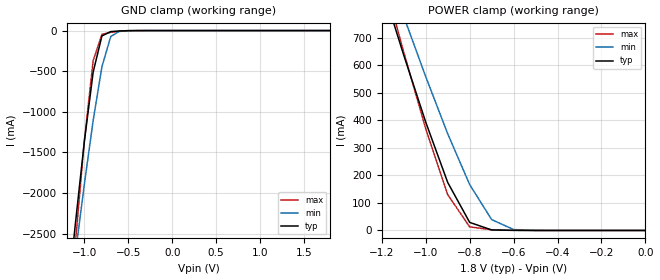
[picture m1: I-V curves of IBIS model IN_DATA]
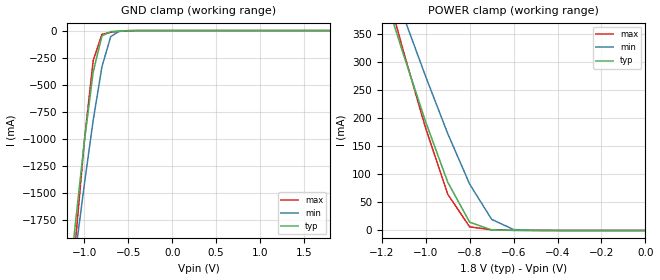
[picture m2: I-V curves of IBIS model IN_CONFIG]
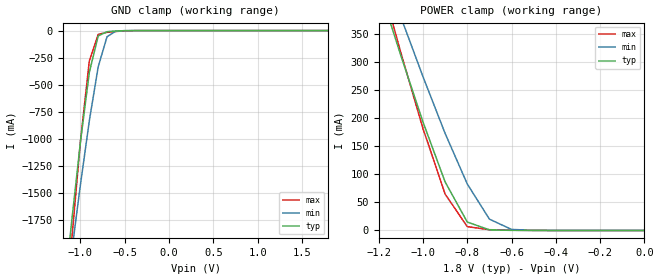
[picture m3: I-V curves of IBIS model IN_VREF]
| IBIS file 4pw864dy_ab_t.ibs created by s2ibis2 version 1.2
| North Carolina State University Electronics Research Laboratory  1995
[IBIS ver]   2.1
[File name]   4pw864dy_ab_t.ibs
[File Rev]   1.0
[Date]   Friday, March 12, 2004
[Source]   IDT
[Notes]   1. Temp typ=25C, min=0C, max=110C
   2. IDT C11.5 1.8V 1P 2-6M process
   3. Ramp rates based on 10Gig ohm load
   *** Important Notes ***
This IBIS file is for the 1:2 Registered Buffer with configuration settings
c0=0, c1=1 (Type A) and c0=1, c1=1 (Type B)
[Disclaimer]
READ THESE TERMS AND CONDITIONS CAREFULLY BEFORE USING THIS IBIS MODEL.  BY
USING THIS IBIS MODEL, YOU ARE ACCEPTING AND AGREEING TO THESE TERMS AND
CONDITIONS OF USE.
Integrated Device Technology, Inc. ("IDT") hereby grants the user of this
IBIS model ("User") a non-exclusive, nontransferable license to use this
IBIS model under the following terms: The User is granted this license only
to use the IBIS model for demonstration purposes only and is not granted
rights to sell, copy (except as needed to run the IBIS model), rent, lease
or sub-license (except for demonstration) the IBIS model in whole or in
part, or in modified form to anyone. The User may modify the IBIS model to
suit its specific applications, but  rights to derivative works and such
modifications shall belong to IDT.
THIS IBIS MODEL IS PROVIDED ON AN AS IS" BASIS AND IDT  MAKES ABSOLUTELY NO
WARRANTY WITH RESPECT TO THE INFORMATION CONTAINED HEREIN.  IDT DISCLAIMS
AND USER WAIVES ALL WARRANTIES, EXPRESS AND IMPLIED, INCLUDING WARRANTIES OF
MERCHANTABILITY AND FITNESS FOR A PARTICULAR PURPOSE.  THE ENTIRE RISK AS TO
QUALITY AND PERFORMANCE IS WITH THE USER  ACCORDINGLY, IN NO EVENT SHALL IDT
BE LIABLE FOR ANY DIRECT OR INDIRECT DAMAGES, WHETHER IN CONTRACT OR TORT,
INCLUDING ANY LOST PROFITS OR OTHER INCIDENTAL, CONSEQUENTIAL, EXEMPLARY, OR
PUNITIVE DAMAGES ARISING OUT OF THE USE OR APPLICATION OF THE  IBIS MODEL,
WHETHER OR NOT IDT HAD NOTICE OF SUCH DAMAGES.
IDT reserves the right to make changes without notice to any product herein
to improve reliability, function, or design. IDT does not convey any license
under patent rights or any other intellectual property rights, including
those of third parties. IDT is not obligated to provide  maintenance or
support for the licensed IBIS model.
This model is IDT74SSTU32864C 1:2 Registered Buffer with 1.8 SSTL I/O
[Copyright]
Copyright 2002, Integrated Device Technology, Inc. All rights
reserved.
|   Component IDT4PW864DY
[Component]   IDT4PW864DY
[Manufacturer]   Integrated Device Technology, Inc.
[Package]
| variable   typ   min   max
R_pkg   0.01480   0.01480   0.01480
L_pkg   1.05000nH   1.05000nH   1.05000nH
C_pkg   0.29100pF   0.29100pF   0.29100pF
[Pin]  signal_name   model_name   R_pin   L_pin   C_pin
A1   DCKE/D1   IN_DATA
A2   NC   NC
A3   VREF   IN_VREF
A4   VDD   POWER
A5   QCKEA/Q1A   OUTBUF
A6   QCKEB/Q1B   OUTBUF
B1   D2   IN_DATA
B2   NC   NC
B3   GND   GND
B4   GND   GND
B5   Q2A   OUTBUF
B6   Q2B   OUTBUF
C1   D3   IN_DATA
C2   NC   NC
C3   VDD   POWER
C4   VDD   POWER
C5   Q3A   OUTBUF
C6   Q3B   OUTBUF
D1   DODT/D4   IN_DATA
D2   NC   NC
D3   GND   GND
D4   GND   GND
D5   QODTA/Q4A   OUTBUF
D6   QODTB/Q4B   OUTBUF
E1   D5   IN_DATA
E2   NC   NC
E3   VDD   POWER
E4   VDD   POWER
E5   Q5A   OUTBUF
E6   Q5B   OUTBUF
F1   D6   IN_DATA
F2   NC   NC
F3   GND   GND
F4   GND   GND
F5   Q6A   OUTBUF
F6   Q6B   OUTBUF
G1   NC   NC
G2   _RESET_   IN_RESET
G3   VDD   POWER
G4   VDD   POWER
G5   C1   IN_CONFIG
G6   C0   IN_CONFIG
H1   CLK   IN_CLK
H2   _DCS_   IN_CSGATEN
H3   GND   GND
H4   GND   GND
H5   _QCSA_   OUTBUF
H6   _QCSB_   OUTBUF
J1   _CLK_   IN_CLK
J2   _CSR_   IN_CSGATEN
J3   VDD   POWER
J4   VDD   POWER
J5   NC   NC
J6   NC   NC
K1   D8   IN_DATA
K2   NC   NC
K3   GND   GND
K4   GND   GND
K5   Q8A   OUTBUF
K6   Q8B   OUTBUF
L1   D9   IN_DATA
L2   NC   NC
L3   VDD   POWER
L4   VDD   POWER
L5   Q9A   OUTBUF
L6   Q9B   OUTBUF
M1   D10   IN_DATA
M2   NC   NC
M3   GND   GND
M4   GND   GND
M5   Q10A   OUTBUF
M6   Q10B   OUTBUF
N1   D11/DODT   IN_DATA
N2   NC   NC
N3   VDD   POWER
N4   VDD   POWER
N5   Q11A/QODTA   OUTBUF
N6   Q11B/QODTB   OUTBUF
P1   D12   IN_DATA
P2   NC   NC
P3   GND   GND
P4   GND   GND
P5   Q12A   OUTBUF
P6   Q12B   OUTBUF
R1   D13   IN_DATA
R2   NC   NC
R3   VDD   POWER
R4   VDD   POWER
R5   Q13A   OUTBUF
R6   Q13B   OUTBUF
T1   D14/DCKE   IN_DATA
T2   NC   NC
T3   VREF   IN_VREF
T4   VDD   POWER
T5   Q14A/QCKEA   OUTBUF
T6   Q14B/QCKEB   OUTBUF
| d   d   dummy_model
| din  din   dummy_model
[Diff Pin]  inv_pin   vdiff   tdelay_typ  tdelay_min  tdelay_max
H1   J1   0.60000V  NA   |CLK<P:N> Input  Pair
| Models and submodels in the file (7): IN_DATA (Input), IN_CONFIG (Input), IN_VREF (Input), IN_CLK (Input), IN_CSGATEN (Input), IN_RESET (Input), OUTBUF (Output)
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|   Model IN_DATA
[Model]   IN_DATA
Model_type   Input
Vinl =  0.65000V
Vinh =  1.15000V
C_comp   2.50000pF   2.50000pF   2.50000pF
[Temperature Range]   25.00000   0.11000k   0.000
[Voltage Range]   1.80000V   1.70000V   1.90000V
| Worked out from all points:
|   GND clamp passes 1 mA (typ) near -0.50 V on its own axis
|   POWER clamp passes 1 mA (typ) near -0.64 V on its own axis
[GND_clamp]
| voltage   I(typ)   I(min)   I(max)
-1.8V     -10.01A    -9.034A    -12.29A
-1.2V     -3.402A    -3.598A    -3.91A
-1.1V     -2.357A    -2.731A    -2.591A
-1V       -1.366A    -1.893A    -1.357A
-900mV    -512.4mA   -1.108A    -371.9mA
-800mV    -65.6mA    -445.2mA   -46.17mA
-700mV    -12.81mA   -74.32mA   -21.4mA
-600mV    -4.632mA   -6.378mA   -10.47mA
-400mV    -151.1uA   -107.5uA   -515.4uA
1.8V      13.82nA    12.76nA    492.7pA
[POWER_clamp]
| voltage   I(typ)   I(min)   I(max)
-1.8V     2.486A     2.403A     2.783A
-1.2V     891mA      1.002A     940.1mA
-1.1V     637mA      777.5mA    647.6mA
-1V       393.6mA    558.9mA    369.7mA
-900mV    174.5mA    351.3mA    130.1mA
-800mV    29.33mA    166.7mA    13.12mA
-700mV    1.951mA    39.57mA    2.484mA
-600mV    305.6uA    3.357mA    798.8uA
-500mV    48.35uA    239.3uA    163.9uA
0V        857.4pA    662pA      637.7pA
|   Model IN_CONFIG
[Model]   IN_CONFIG
Model_type   Input
Vinl =  0.000V
Vinh =  1.80000V
C_comp   1.750000pF   1.75000pF   1.75000pF
[Temperature Range]   25.00000   0.11000k   0.000
[Voltage Range]   1.80000V   1.70000V   1.90000V
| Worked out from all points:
|   GND clamp passes 1 mA (typ) near -0.51 V on its own axis
|   POWER clamp passes 1 mA (typ) near -0.70 V on its own axis
[GND_clamp]
| voltage   I(typ)   I(min)   I(max)
-1.8V     -7.509A    -6.777A    -9.219A
-1.2V     -2.552A    -2.699A    -2.933A
-1.1V     -1.768A    -2.049A    -1.943A
-1V       -1.025A    -1.42A     -1.018A
-900mV    -384.3mA   -831.8mA   -278.9mA
-800mV    -49.16mA   -334.1mA   -34.6mA
-700mV    -9.52mA    -55.82mA   -15.97mA
-600mV    -3.358mA   -4.767mA   -7.725mA
-400mV    -53.67uA   -34.09uA   -242.5uA
1.8V      26.95pA    5.248nA    -19.88pA
[POWER_clamp]
| voltage   I(typ)   I(min)   I(max)
-1.8V     1.209A     1.169A     1.353A
-1.2V     434.4mA    488.7mA    458.3mA
-1.1V     311.1mA    379.5mA    316.3mA
-1V       192.7mA    273.3mA    181mA
-900mV    85.9mA     172.3mA    64.37mA
-800mV    14.67mA    82.28mA    6.452mA
-700mV    926.3uA    19.77mA    1.156mA
-600mV    137.1uA    1.636mA    359.6uA
-500mV    21.08uA    107.7uA    70.28uA
0V        26.95pA    124.4pA    8.257pA
|   Model IN_VREF
[Model]   IN_VREF
Model_type   Input
Vinl =  0.83300V
Vinh =  0.96900V
C_comp   1.750000pF   1.75000pF   1.75000pF
[Temperature Range]   25.00000   0.11000k   0.000
[Voltage Range]   1.80000V   1.70000V   1.90000V
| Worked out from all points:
|   GND clamp passes 1 mA (typ) near -0.50 V on its own axis
|   POWER clamp passes 1 mA (typ) near -0.69 V on its own axis
[GND_clamp]
| voltage   I(typ)   I(min)   I(max)
-1.8V     -7.51A     -6.777A    -9.22A
-1.2V     -2.552A    -2.7A      -2.934A
-1.1V     -1.768A    -2.049A    -1.944A
-1V       -1.025A    -1.42A     -1.018A
-900mV    -385mA     -832.1mA   -279.5mA
-800mV    -49.71mA   -334.4mA   -35.16mA
-700mV    -10.01mA   -56.13mA   -16.48mA
-600mV    -3.774mA   -5.075mA   -8.176mA
-300mV    -47.02uA   -56.45uA   -126.6uA
1.8V      49.15nA    26.41nA    5.103nA
[POWER_clamp]
| voltage   I(typ)   I(min)   I(max)
-1.8V     1.213A     1.173A     1.357A
-1.2V     436.1mA    490.7mA    459.9mA
-1.1V     312.4mA    381.2mA    317.5mA
-1V       193.7mA    274.6mA    182mA
-900mV    86.67mA    173.3mA    64.98mA
-800mV    15.07mA    83.05mA    6.858mA
-700mV    1.114mA    20.26mA    1.39mA
-600mV    207.8uA    1.878mA    482.9uA
-500mV    38.54uA    180.7uA    114.2uA
0V        5.276nA    15.76nA    22.22nA
